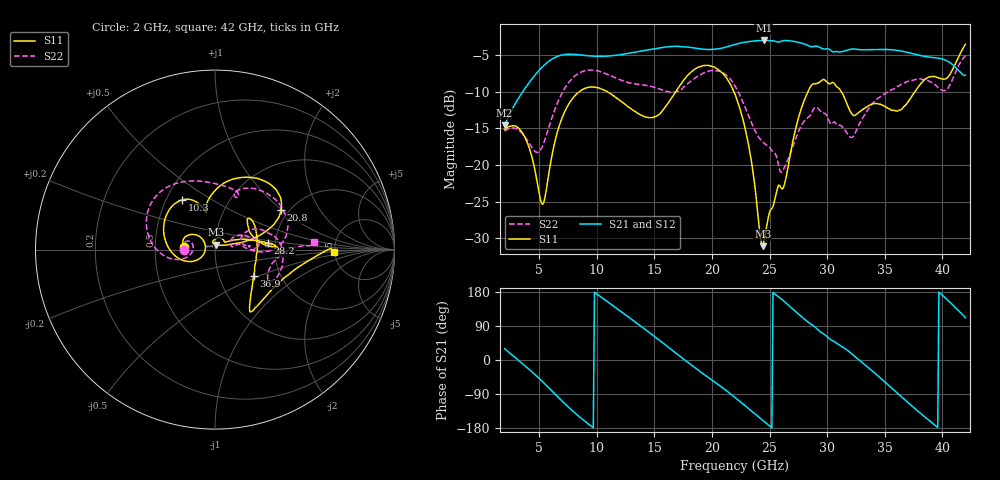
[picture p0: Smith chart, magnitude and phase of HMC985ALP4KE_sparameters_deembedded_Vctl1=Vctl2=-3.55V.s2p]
!s2p File: Measurements: S11, S21, S12, S22
# GHz S dB R 50.0
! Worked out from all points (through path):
!   401 points, 2 GHz to 42 GHz, reference 50 ohm
!   highest |S21| = -3.03 dB at 24.5 GHz (marker M1); lowest = -14.6 dB at 2 GHz (marker M2)
!   lowest |S11| = -31.0 dB at 24.4 GHz (marker M3), VSWR 1.06, Z = 50.5 + j2.78 ohm
!   |S11| at or under -10 dB: start of sweep to 8.487 GHz; 21.9 GHz to 28.34 GHz (6.441 GHz wide, 25.6 % of centre); 31.23 GHz to 37.63 GHz (6.406 GHz wide, 18.6 % of centre)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
!   |S22| runs from -21.0 to -5.1 dB; largest |S21 - S12| = 0.00061
!   S11 on the Smith chart (normalised r, x): 2 GHz: 0.70, +0.02; 10.3 GHz: 0.60, +0.37; 20.8 GHz: 1.82, +0.99; 28.2 GHz: 1.84, +0.15; 36.9 GHz: 1.46, -0.46; 42 GHz: 4.96, -0.26
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2  -15.15 175.6  -14.61 29.9  -14.62 29.9  -15.39 -179.6
3.7  -16.04 147.7  -9.72 -13.3  -9.72 -13.3  -16.04 162.4
5.3  -25.34 176.1  -6.60 -57.3  -6.60 -57.3  -17.39 -170.9
6.9  -13.93 -164.5  -5.04 -105.8  -5.04 -105.8  -10.45 -175.5
8.7  -9.77 149.7  -5.03 -155.0  -5.03 -155.0  -7.29 149.8
10.3  -9.58 123.7  -5.20 167.7  -5.20 167.7  -7.28 123.5
13.2  -12.57 105.0  -4.67 103.4  -4.67 103.4  -8.90 82.1
15.4  -13.12 103.3  -4.07 53.1  -4.07 53.1  -9.62 66.4
17.8  -7.94 76.7  -3.92 -3.7  -3.92 -3.8  -9.04 69.0
20.8  -7.33 31.1  -4.10 -70.5  -4.11 -70.5  -7.29 20.5
22  -10.36 19.8  -3.58 -98.8  -3.58 -98.8  -9.22 2.1
23.2  -17.44 15.8  -3.19 -128.7  -3.19 -128.7  -13.38 -1.8
24.4  -31.05 78.8  -3.04 -158.9  -3.03 -158.8  -16.86 10.9
24.5  -30.44 90.2  -3.03 -161.4  -3.03 -161.4  -16.98 11.7
26.1  -23.26 37.7  -3.08 159.3  -3.08 159.3  -20.88 23.0
28.2  -10.49 7.0  -3.62 103.5  -3.62 103.5  -13.71 18.6
28.7  -9.01 0.6  -3.89 92.6  -3.89 92.6  -12.73 15.2
32.4  -13.25 28.6  -4.21 9.3  -4.20 9.3  -15.76 25.2
35.4  -12.35 13.3  -4.28 -68.6  -4.27 -68.6  -9.96 15.9
36.9  -11.67 -34.6  -4.63 -109.2  -4.63 -109.2  -8.65 3.9
39.6  -8.10 -54.8  -5.43 -178.2  -5.43 -178.2  -9.41 -29.4
42  -3.54 -1.3  -7.78 111.2  -7.79 111.2  -5.11 4.2
